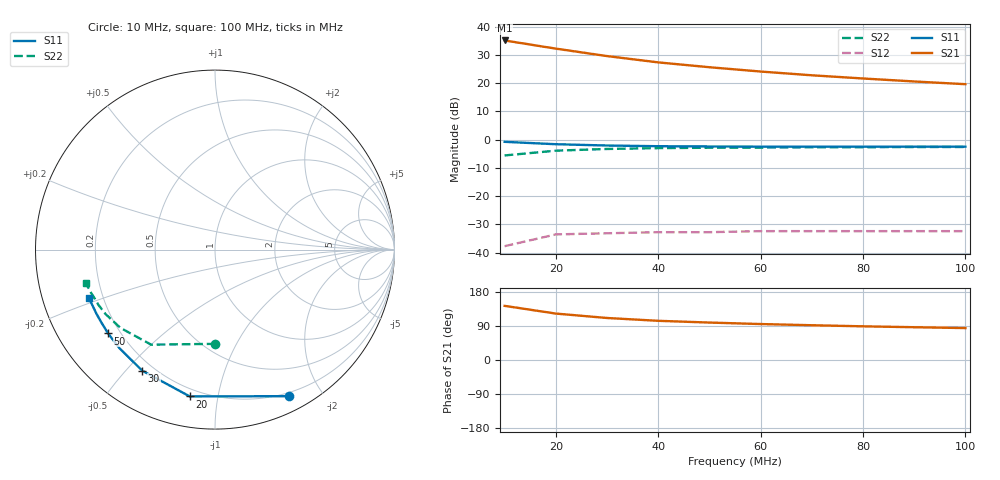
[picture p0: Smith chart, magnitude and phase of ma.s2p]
# MHZ  S  MA  R  50
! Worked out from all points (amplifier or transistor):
!   10 points, 10 MHz to 100 MHz, reference 50 ohm
!   highest |S21| = 35.1 dB at 10 MHz (marker M1)
!   |S21| within 3 dB of that: start of sweep to 20.4 MHz
!   unconditionally stable (mu >= 1): nowhere
!   at 20 MHz: K = 0.03, MSG = 32.9 dB, |S12| = -33.6 dB
!   at 60 MHz: K = 0.09, MSG = 28.3 dB, |S12| = -32.4 dB
!   at 100 MHz: K = 0.15, MSG = 26.0 dB, |S12| = -32.4 dB
!   S11 on the Smith chart (normalised r, x): 10 MHz: 0.16, -1.61; 20 MHz: 0.16, -0.83; 30 MHz: 0.16, -0.56; 50 MHz: 0.15, -0.34; 100 MHz: 0.15, -0.18
10  0.915 -63.2  57.03 142.9  0.013 51.9  0.525 -89.7
20  0.83 -99.8  40.87 122.5  0.021 32.5  0.638 -123.9
30  0.787 -121.0  30.18 110.9  0.022 20.8  0.684 -140.4
40  0.765 -134.1  23.33 103.4  0.023 15.2  0.708 -149.6
50  0.757 -141.9  19.15 98.8  0.023 10.4  0.719 -154.7
60  0.752 -147.4  16.06 94.9  0.024 5.9  0.724 -158.2
70  0.751 -151.5  13.79 91.7  0.024 2.8  0.732 -160.9
80  0.75 -154.6  12.1 88.9  0.024 2.8  0.735 -162.6
90  0.751 -156.7  10.72 86.5  0.024 -0.8  0.74 -164.2
100  0.75 -159.0  9.593 84.3  0.024 -3.2  0.742 -165.3
